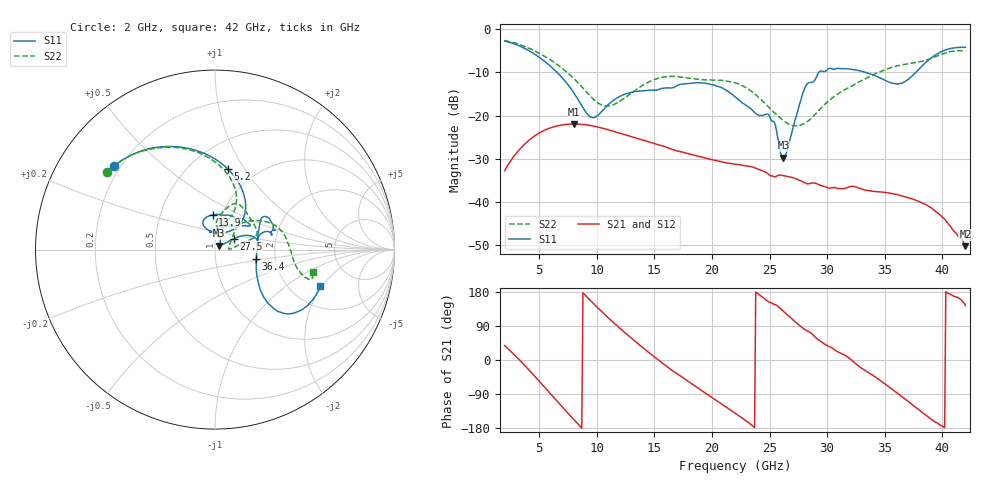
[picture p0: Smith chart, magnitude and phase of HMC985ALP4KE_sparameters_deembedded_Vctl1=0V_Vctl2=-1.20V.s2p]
!s2p File: Measurements: S11, S21, S12, S22
# GHz S dB R 50.0
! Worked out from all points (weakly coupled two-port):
!   401 points, 2 GHz to 42 GHz, reference 50 ohm
!   highest |S21| = -21.97 dB at 8 GHz (marker M1); lowest = -50.3 dB at 42 GHz (marker M2)
!   lowest |S11| = -29.8 dB at 26.2 GHz (marker M3), VSWR 1.07, Z = 52.4 + j2.28 ohm
!   |S11| at or under -10 dB: 6.557 GHz to 29.27 GHz (22.71 GHz wide, 127 % of centre); 33.35 GHz to 37.69 GHz (4.344 GHz wide, 12.2 % of centre)
!   |S22| runs from -22.4 to -2.6 dB; largest |S21 - S12| = 0.00014
!   S11 on the Smith chart (normalised r, x): 2 GHz: 0.17, +0.35; 5.2 GHz: 0.75, +0.84; 13.9 GHz: 0.90, +0.36; 27.5 GHz: 1.22, +0.15; 36.4 GHz: 1.58, -0.18; 42 GHz: 2.90, -1.91
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2  -2.72 140.4  -32.79 38.0  -32.78 37.9  -2.58 144.2
3.5  -4.12 112.7  -27.28 -6.4  -27.28 -6.4  -3.73 119.5
5.2  -6.87 80.7  -23.76 -62.7  -23.77 -62.7  -5.85 93.5
8  -14.69 45.9  -21.97 -157.0  -21.97 -157.0  -11.39 64.5
8.7  -17.75 51.9  -22.05 -179.6  -22.05 -179.6  -13.34 63.6
9.7  -20.49 85.3  -22.44 149.3  -22.44 149.3  -16.18 69.4
10.9  -17.71 113.5  -23.22 114.0  -23.22 114.0  -17.79 83.3
13.9  -14.25 93.9  -25.61 34.9  -25.60 34.9  -13.13 77.4
15.4  -13.94 73.0  -26.83 -0.9  -26.83 -1.0  -11.29 68.4
19.4  -12.52 34.5  -29.84 -86.6  -29.85 -86.6  -11.71 36.7
22  -15.62 52.3  -31.27 -139.8  -31.28 -139.8  -12.40 18.5
25  -20.17 98.0  -33.84 152.3  -33.84 152.2  -18.26 9.2
26.2  -29.80 42.1  -33.93 128.2  -33.93 128.1  -21.18 1.9
27.5  -18.39 29.8  -34.91 93.6  -34.90 93.4  -22.34 6.2
28.1  -13.35 20.8  -35.63 79.7  -35.65 79.5  -21.73 15.5
28.7  -12.31 12.9  -35.65 68.4  -35.64 68.3  -20.40 25.2
31  -9.08 23.3  -36.93 20.7  -36.92 20.5  -14.84 45.7
33.3  -9.96 34.4  -37.30 -27.5  -37.28 -27.3  -11.49 37.0
35.4  -12.27 12.3  -37.97 -71.7  -37.98 -71.8  -9.05 23.3
36.4  -12.57 -12.8  -38.58 -94.7  -38.60 -94.9  -8.27 15.7
39.5  -5.80 -43.3  -42.47 -165.3  -42.41 -165.8  -6.22 -14.4
42  -4.14 -19.0  -50.29 143.7  -50.04 144.3  -5.03 -13.0
